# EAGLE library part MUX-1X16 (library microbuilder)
1x16 Channel Analog Multiplexer/Demultiplexer [Part No.] Texas Instruments CD74HC4067 Digikey: 296-9226-6-ND
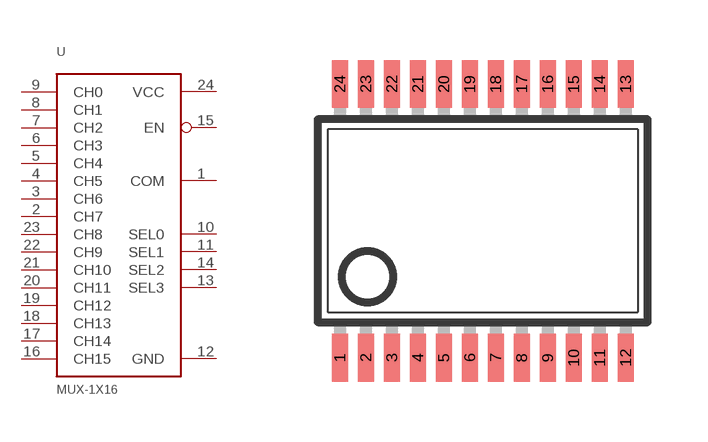
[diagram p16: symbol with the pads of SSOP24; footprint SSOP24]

Designator prefix U

## MUX-1X16  [SSOP24]
1  COM
2  CH7
3  CH6
4  CH5
5  CH4
6  CH3
7  CH2
8  CH1
9  CH0
10  SEL0
11  SEL1
12  GND
13  SEL3
14  SEL2
15  EN
16  CH15
17  CH14
18  CH13
19  CH12
20  CH11
21  CH10
22  CH9
23  CH8
24  VCC

## Footprint SSOP24 (pad centres in mm)
Small Shrink Outline Package SOT340-1 / JEDEC MO-150AG
smd 0.4 x 1.2: 1 -3.575,-3.42; 2 -2.925,-3.42; 3 -2.275,-3.42; 4 -1.625,-3.42; 5 -0.975,-3.42; 6 -0.325,-3.42; 7 0.325,-3.42; 8 0.975,-3.42; 9 1.625,-3.42; 10 2.275,-3.42; 11 2.925,-3.42; 12 3.575,-3.42; 13 3.575,3.42; 14 2.925,3.42; 15 2.275,3.42; 16 1.625,3.42; 17 0.975,3.42; 18 0.325,3.42; 19 -0.325,3.42; 20 -0.975,3.42; 21 -1.625,3.42; 22 -2.275,3.42; 23 -2.925,3.42; 24 -3.575,3.42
